| IBIS file stm32u575_585_ufbga169.ibs
[IBIS ver] 4.2
[File name] stm32u575_585_ufbga169.ibs
[File Rev] 1.0
[Date]   06-08-2021
[Source] Data Created at STMicroelectronics
[Notes]  File originated from ELDO simulations.
[Disclaimer]  This information is for modeling purpose only and is
   not guaranted. The information is subject to change without
   notice.
[Copyright] Copyright 2021 STMicroelectronics Inc.
|   Component stm32u575_585_ufbga169
[Component] stm32u575_585_ufbga169
[Manufacturer] STMicroelectronics
[Package]
| variable   typ   min   max
R_pkg   0   NA   NA
L_pkg   0   NA   NA
C_pkg   0   NA   NA
[Pin]   signal_name   model_name   R_pin   L_pin   C_pin   | Comment
A1 PE2 io8_100m_hslv_ft
A10 PA15 nc
A11 VDD POWER
A12 PI1 io8_100m_hslv_ft
A13 PH15 io8_100m_hslv_ft
A2 PI6 io8_166m_hslv_ft
A3 VDD POWER
A4 VCAP POWER
A5 PG15 io8_100m_hslv_ft
A6 VDDIO2 POWER
A7 PG9 io8_100m_hslv_ft
A8 VDD POWER
A9 PC11 io8_100m_hslv_ft
B1 VDD POWER
B10 PI4 io8_100m_ft
B11 VSS GND
B12 PI0 io8_100m_hslv_ft
B13 PH12 io8_100m_hslv_ft
B2 VSS GND
B3 PI5 io8_100m_hslv_ft
B4 VSS GND
B5 PB6 io8_100m_i2c_ft
B6 PB4 io8_100m_i2c_ft
B7 PD6 io8_166m_hslv_ft
B8 VSS GND
B9 PD0 io8_100m_hslv_ft
C1 VBAT POWER
C10 PA14 io8_100m_ft
C11 PH14 io8_100m_ft
C12 PH13 io8_100m_ft
C13 PH10 io8_100m_hslv_ft
C2 PE4 io8_100m_hslv_tamp_ft
C3 PI7 io8_166m_hslv_ft
C4 PE1 io8_100m_hslv_ft
C5 PH3-BOOT0 io8_100m_ft
C6 PB5 io8_166m_hslv_ft
C7 PG10 io8_100m_hslv_ft
C8 PD4 io8_100m_hslv_ft
C9 PC10 io8_100m_ft
D1 PC14-OSC32_IN io8_100m_ft
D10 PI3 io8_100m_hslv_ft
D11 PI2 io8_166m_hslv_ft
D12 PH8 io8_100m_hslv_ft
D13 VDD POWER
D2 PE5 io8_100m_hslv_tamp_ft
D3 PE3 io8_100m_hslv_tamp_ft
D4 PE0 io8_100m_hslv_ft
D5 PB9 io8_100m_i2c_ft
D6 PB3 io8_100m_i2c_ft
D7 PD7 io8_100m_hslv_ft
D8 PD3 io8_166m_hslv_ft
D9 PH11 io8_100m_hslv_ft
E1 PC15-OSC32_OUT io8_100m_ft
E10 PH4 io8_100m_hslv_ft
E11 PH6 io8_166m_hslv_ft
E12 VSS GND
E13 VDDUSB POWER
E2 PF0 io8_100m_hslv_ft
E3 PC13 io8_100m_ft_v33
E4 PE6 io8_100m_hslv_tamp_ft
E5 PB8 io8_100m_i2c_ft
E6 PG12 io8_100m_hslv_ft
E7 PD5 io8_100m_hslv_ft
E8 PC12 io8_166m_hslv_ft
E9 PH9 io8_100m_hslv_ft
F1 PF8 io8_100m_hslv_ft
F10 PH2 io8_100m_hslv_ft
F11 PA10 io8_100m_usb_id
F12 PA13 io8_100m_ft
F13 PA12 io8_usb_ft
F2 VSS GND
F3 PF1 io8_100m_hslv_ft
F4 PF2 io8_100m_hslv_ft
F5 PB7 io8_166m_hslv_i2c_ft
F6 PD1 io8_100m_hslv_ft
F7 PD2 io8_100m_ft
F8 PH7 io8_166m_hslv_i2c_ft
F9 PH5 io8_100m_i2c_ft
G1 VDD POWER
G10 PC8 io8_100m_ft
G11 PA9 io8_100m_usb_vbus_ft
G12 PC7 io8_100m_ft
G13 PA11 io8_usb_ft
G2 PF7 io8_100m_hslv_ft
G3 PF9 io8_100m_hslv_ft
G4 PF5 io8_166m_hslv_ft
G5 PF3 io8_100m_hslv_ft
G6 PF4 io8_166m_hslv_ft
G7 PA8 io8_166m_hslv_ft
G8 PG7 io8_100m_hslv_ft
G9 PC9 io8_100m_ft
H1 PH0-OSC_IN io8_100m_ft
H10 PG6 io8_100m_hslv_ft
H11 PG4 io8_100m_hslv_ft
H12 VDDIO2 POWER
H13 PC6 io8_100m_ft
H2 VSS GND
H3 NRST nc
H4 PF10 io8_166m_hslv_ft
H5 OPAMP2_VINM nc
H6 PF6 io8_100m_hslv_ft
H7 PG1 io8_100m_hslv_ft
H8 PE10 io8_166m_hslv_ft
H9 PG8 io8_100m_i2c_ft
J1 PH1-OSC_OUT io8_100m_ft
J10 PD14 io8_100m_hslv_ft
J11 PD15 io8_100m_hslv_ft
J12 VSS GND
J13 VDD POWER
J2 PC0 io8_100m_hslv_ft
J3 PC1 io8_166m_hslv_i2c_ft
J4 PC2 io8_100m_hslv_ft
J5 PA7 io8_100m_hslv_ft
J6 PG0 io8_100m_hslv_ft
J7 PE9 io8_166m_hslv_ft
J8 PG3 io8_100m_hslv_ft
J9 PG5 io8_100m_hslv_ft
K1 PC3 io8_100m_hslv_ft
K10 PD12 io8_100m_hslv_ft
K11 PD10 io8_100m_hslv_ft
K12 PD13 io8_100m_hslv_ft
K13 PG2 io8_100m_hslv_ft
K2 VSSA GND
K3 PA0 io8_100m_hslv_tamp_ft
K4 PA5 io8_100m_ft
K5 PB0 io8_100m_hslv_ft
K6 PF12 io8_100m_hslv_ft
K7 PE8 io8_100m_hslv_ft
K8 PE14 io8_100m_hslv_ft
K9 PB10 io8_166m_hslv_i2c_ft
L1 VREF+ POWER
L10 PB12 io8_166m_hslv_ft
L11 PB15 nc
L12 PD8 io8_100m_hslv_ft
L13 PD9 io8_100m_hslv_ft
L2 VDDA POWER
L3 PA1 io8_100m_hslv_tamp_ft
L4 PC4 io8_100m_hslv_ft
L5 PB2 io8_100m_hslv_tamp_ft
L6 PF14 io8_100m_hslv_ft
L7 PE7 io8_100m_hslv_ft
L8 PE13 io8_100m_hslv_ft
L9 PB11 io8_100m_hslv_ft
M1 OPAMP1_VINM nc
M10 PG11 io8_100m_hslv_ft
M11 VSS GND
M12 PB14 io8_100m_i2c_ft
M13 PD11 io8_100m_hslv_ft
M2 PA2 io8_100m_hslv_ft
M3 VSS GND
M4 PC5 io8_100m_tamp_ft
M5 PF11 io8_166m_hslv_ft
M6 PF13 io8_100m_hslv_ft
M7 VSS GND
M8 PE11 io8_100m_hslv_ft
M9 PE15 io8_100m_hslv_ft
N1 PA4 io8_100m_hslv_ft
N10 PG13 io8_100m_hslv_ft
N11 VCAP POWER
N12 VDD POWER
N13 PB13 io8_100m_i2c_ft
N2 PA3 io8_166m_hslv_ft
N3 VDD POWER
N4 PA6 io8_100m_hslv_ft
N5 PB1 io8_100m_hslv_ft
N6 PF15 io8_100m_hslv_ft
N7 VDD POWER
N8 PE12 io8_100m_hslv_ft
N9 PG14 io8_100m_hslv_ft
[Model Selector] io8_100m_ft
io8_100m_ft_hs_1v2  "IO8_FT 100MHz high speed @ 1.2V"
io8_100m_ft_hs_pu_1v2  "IO8_FT 100MHz high speed @ 1.2V pullup"
io8_100m_ft_hs_pd_1v2  "IO8_FT 100MHz high speed @ 1.2V pulldown"
io8_100m_ft_fs_1v2  "IO8_FT 100MHz fast speed @ 1.2V"
io8_100m_ft_fs_pu_1v2  "IO8_FT 100MHz fast speed @ 1.2V pullup"
io8_100m_ft_fs_pd_1v2  "IO8_FT 100MHz fast speed @ 1.2V pulldown"
io8_100m_ft_ms_1v2  "IO8_FT 100MHz med speed @ 1.2V"
io8_100m_ft_ms_pu_1v2  "IO8_FT 100MHz med speed @ 1.2V pullup"
io8_100m_ft_ms_pd_1v2  "IO8_FT 100MHz med speed @ 1.2V pulldown"
io8_100m_ft_ls_1v2  "IO8_FT 100MHz low speed @ 1.2V"
io8_100m_ft_ls_pu_1v2  "IO8_FT 100MHz low speed @ 1.2V pullup"
io8_100m_ft_ls_pd_1v2  "IO8_FT 100MHz low speed @ 1.2V pulldown"
io8_100m_ft_hs_1v8  "IO8_FT 100MHz high speed @ 1.8V"
io8_100m_ft_hs_pu_1v8  "IO8_FT 100MHz high speed @ 1.8V pullup"
io8_100m_ft_hs_pd_1v8  "IO8_FT 100MHz high speed @ 1.8V pulldown"
io8_100m_ft_fs_1v8  "IO8_FT 100MHz fast speed @ 1.8V"
io8_100m_ft_fs_pu_1v8  "IO8_FT 100MHz fast speed @ 1.8V pullup"
io8_100m_ft_fs_pd_1v8  "IO8_FT 100MHz fast speed @ 1.8V pulldown"
io8_100m_ft_ms_1v8  "IO8_FT 100MHz med speed @ 1.8V"
io8_100m_ft_ms_pu_1v8  "IO8_FT 100MHz med speed @ 1.8V pullup"
io8_100m_ft_ms_pd_1v8  "IO8_FT 100MHz med speed @ 1.8V pulldown"
io8_100m_ft_ls_1v8  "IO8_FT 100MHz low speed @ 1.8V"
io8_100m_ft_ls_pu_1v8  "IO8_FT 100MHz low speed @ 1.8V pullup"
io8_100m_ft_ls_pd_1v8  "IO8_FT 100MHz low speed @ 1.8V pulldown"
io8_100m_ft_hs_3v3  "IO8_FT 100MHz high speed @ 3.3V"
io8_100m_ft_hs_pu_3v3  "IO8_FT 100MHz high speed @ 3.3V pullup"
io8_100m_ft_hs_pd_3v3  "IO8_FT 100MHz high speed @ 3.3V pulldown"
io8_100m_ft_fs_3v3  "IO8_FT 100MHz fast speed @ 3.3V"
io8_100m_ft_fs_pu_3v3  "IO8_FT 100MHz fast speed @ 3.3V pullup"
io8_100m_ft_fs_pd_3v3  "IO8_FT 100MHz fast speed @ 3.3V pulldown"
io8_100m_ft_ms_3v3  "IO8_FT 100MHz med speed @ 3.3V"
io8_100m_ft_ms_pu_3v3  "IO8_FT 100MHz med speed @ 3.3V pullup"
io8_100m_ft_ms_pd_3v3  "IO8_FT 100MHz med speed @ 3.3V pulldown"
io8_100m_ft_ls_3v3  "IO8_FT 100MHz low speed @ 3.3V"
io8_100m_ft_ls_pu_3v3  "IO8_FT 100MHz low speed @ 3.3V pullup"
io8_100m_ft_ls_pd_3v3  "IO8_FT 100MHz low speed @ 3.3V pulldown"
[Model Selector] io8_100m_hslv_ft
io8_100m_ft_hs_1v2  "IO8_FT 100MHz high speed @ 1.2V"
io8_100m_ft_hs_pu_1v2  "IO8_FT 100MHz high speed @ 1.2V pullup"
io8_100m_ft_hs_pd_1v2  "IO8_FT 100MHz high speed @ 1.2V pulldown"
io8_100m_ft_fs_1v2  "IO8_FT 100MHz fast speed @ 1.2V"
io8_100m_ft_fs_pu_1v2  "IO8_FT 100MHz fast speed @ 1.2V pullup"
io8_100m_ft_fs_pd_1v2  "IO8_FT 100MHz fast speed @ 1.2V pulldown"
io8_100m_ft_ms_1v2  "IO8_FT 100MHz med speed @ 1.2V"
io8_100m_ft_ms_pu_1v2  "IO8_FT 100MHz med speed @ 1.2V pullup"
io8_100m_ft_ms_pd_1v2  "IO8_FT 100MHz med speed @ 1.2V pulldown"
io8_100m_ft_ls_1v2  "IO8_FT 100MHz low speed @ 1.2V"
io8_100m_ft_ls_pu_1v2  "IO8_FT 100MHz low speed @ 1.2V pullup"
io8_100m_ft_ls_pd_1v2  "IO8_FT 100MHz low speed @ 1.2V pulldown"
io8_100m_ft_hs_1v8  "IO8_FT 100MHz high speed @ 1.8V"
io8_100m_ft_hs_pu_1v8  "IO8_FT 100MHz high speed @ 1.8V pullup"
io8_100m_ft_hs_pd_1v8  "IO8_FT 100MHz high speed @ 1.8V pulldown"
io8_100m_ft_fs_1v8  "IO8_FT 100MHz fast speed @ 1.8V"
io8_100m_ft_fs_pu_1v8  "IO8_FT 100MHz fast speed @ 1.8V pullup"
io8_100m_ft_fs_pd_1v8  "IO8_FT 100MHz fast speed @ 1.8V pulldown"
io8_100m_ft_ms_1v8  "IO8_FT 100MHz med speed @ 1.8V"
io8_100m_ft_ms_pu_1v8  "IO8_FT 100MHz med speed @ 1.8V pullup"
io8_100m_ft_ms_pd_1v8  "IO8_FT 100MHz med speed @ 1.8V pulldown"
io8_100m_ft_ls_1v8  "IO8_FT 100MHz low speed @ 1.8V"
io8_100m_ft_ls_pu_1v8  "IO8_FT 100MHz low speed @ 1.8V pullup"
io8_100m_ft_ls_pd_1v8  "IO8_FT 100MHz low speed @ 1.8V pulldown"
io8_100m_ft_hs_3v3  "IO8_FT 100MHz high speed @ 3.3V"
io8_100m_ft_hs_pu_3v3  "IO8_FT 100MHz high speed @ 3.3V pullup"
io8_100m_ft_hs_pd_3v3  "IO8_FT 100MHz high speed @ 3.3V pulldown"
io8_100m_ft_fs_3v3  "IO8_FT 100MHz fast speed @ 3.3V"
io8_100m_ft_fs_pu_3v3  "IO8_FT 100MHz fast speed @ 3.3V pullup"
io8_100m_ft_fs_pd_3v3  "IO8_FT 100MHz fast speed @ 3.3V pulldown"
io8_100m_ft_ms_3v3  "IO8_FT 100MHz med speed @ 3.3V"
io8_100m_ft_ms_pu_3v3  "IO8_FT 100MHz med speed @ 3.3V pullup"
io8_100m_ft_ms_pd_3v3  "IO8_FT 100MHz med speed @ 3.3V pulldown"
io8_100m_ft_ls_3v3  "IO8_FT 100MHz low speed @ 3.3V"
io8_100m_ft_ls_pu_3v3  "IO8_FT 100MHz low speed @ 3.3V pullup"
io8_100m_ft_ls_pd_3v3  "IO8_FT 100MHz low speed @ 3.3V pulldown"
io8_100m_hslv_ft_hs_1v2  "IO8_FT 100MHz HSLV high speed @ 1.2V"
io8_100m_hslv_ft_hs_pu_1v2  "IO8_FT 100MHz HSLV high speed @ 1.2V pullup"
io8_100m_hslv_ft_hs_pd_1v2  "IO8_FT 100MHz HSLV high speed @ 1.2V pulldown"
io8_100m_hslv_ft_fs_1v2  "IO8_FT 100MHz HSLV fast speed @ 1.2V"
io8_100m_hslv_ft_fs_pu_1v2  "IO8_FT 100MHz HSLV fast speed @ 1.2V pullup"
io8_100m_hslv_ft_fs_pd_1v2  "IO8_FT 100MHz HSLV fast speed @ 1.2V pulldown"
io8_100m_hslv_ft_ms_1v2  "IO8_FT 100MHz HSLV med speed @ 1.2V"
io8_100m_hslv_ft_ms_pu_1v2  "IO8_FT 100MHz HSLV med speed @ 1.2V pullup"
io8_100m_hslv_ft_ms_pd_1v2  "IO8_FT 100MHz HSLV med speed @ 1.2V pulldown"
io8_100m_hslv_ft_ls_1v2  "IO8_FT 100MHz HSLV low speed @ 1.2V"
io8_100m_hslv_ft_ls_pu_1v2  "IO8_FT 100MHz HSLV low speed @ 1.2V pullup"
io8_100m_hslv_ft_ls_pd_1v2  "IO8_FT 100MHz HSLV low speed @ 1.2V pulldown"
io8_100m_hslv_ft_hs_1v8  "IO8_FT 100MHz HSLV high speed @ 1.8V"
io8_100m_hslv_ft_hs_pu_1v8  "IO8_FT 100MHz HSLV high speed @ 1.8V pullup"
io8_100m_hslv_ft_hs_pd_1v8  "IO8_FT 100MHz HSLV high speed @ 1.8V pulldown"
io8_100m_hslv_ft_fs_1v8  "IO8_FT 100MHz HSLV fast speed @ 1.8V"
io8_100m_hslv_ft_fs_pu_1v8  "IO8_FT 100MHz HSLV fast speed @ 1.8V pullup"
io8_100m_hslv_ft_fs_pd_1v8  "IO8_FT 100MHz HSLV fast speed @ 1.8V pulldown"
io8_100m_hslv_ft_ms_1v8  "IO8_FT 100MHz HSLV med speed @ 1.8V"
io8_100m_hslv_ft_ms_pu_1v8  "IO8_FT 100MHz HSLV med speed @ 1.8V pullup"
io8_100m_hslv_ft_ms_pd_1v8  "IO8_FT 100MHz HSLV med speed @ 1.8V pulldown"
io8_100m_hslv_ft_ls_1v8  "IO8_FT 100MHz HSLV low speed @ 1.8V"
io8_100m_hslv_ft_ls_pu_1v8  "IO8_FT 100MHz HSLV low speed @ 1.8V pullup"
io8_100m_hslv_ft_ls_pd_1v8  "IO8_FT 100MHz HSLV low speed @ 1.8V pulldown"
io8_100m_hslv_ft_hs_2v5  "IO8_FT 100MHz HSLV high speed @ 2.5V"
io8_100m_hslv_ft_hs_pu_2v5  "IO8_FT 100MHz HSLV high speed @ 2.5V pullup"
io8_100m_hslv_ft_hs_pd_2v5  "IO8_FT 100MHz HSLV high speed @ 2.5V pulldown"
io8_100m_hslv_ft_fs_2v5  "IO8_FT 100MHz HSLV fast speed @ 2.5V"
io8_100m_hslv_ft_fs_pu_2v5  "IO8_FT 100MHz HSLV fast speed @ 2.5V pullup"
io8_100m_hslv_ft_fs_pd_2v5  "IO8_FT 100MHz HSLV fast speed @ 2.5V pulldown"
io8_100m_hslv_ft_ms_2v5  "IO8_FT 100MHz HSLV med speed @ 2.5V"
io8_100m_hslv_ft_ms_pu_2v5  "IO8_FT 100MHz HSLV med speed @ 2.5V pullup"
io8_100m_hslv_ft_ms_pd_2v5  "IO8_FT 100MHz HSLV med speed @ 2.5V pulldown"
io8_100m_hslv_ft_ls_2v5  "IO8_FT 100MHz HSLV low speed @ 2.5V"
io8_100m_hslv_ft_ls_pu_2v5  "IO8_FT 100MHz HSLV low speed @ 2.5V pullup"
io8_100m_hslv_ft_ls_pd_2v5  "IO8_FT 100MHz HSLV low speed @ 2.5V pulldown"
[Model Selector] io8_166m_hslv_ft
io8_166m_ft_hs_1v2  "IO8_FT 166MHz high speed @ 1.2V"
io8_166m_ft_hs_pu_1v2  "IO8_FT 166MHz high speed @ 1.2V pullup"
io8_166m_ft_hs_pd_1v2  "IO8_FT 166MHz high speed @ 1.2V pulldown"
io8_166m_ft_fs_1v2  "IO8_FT 166MHz fast speed @ 1.2V"
io8_166m_ft_fs_pu_1v2  "IO8_FT 166MHz fast speed @ 1.2V pullup"
io8_166m_ft_fs_pd_1v2  "IO8_FT 166MHz fast speed @ 1.2V pulldown"
io8_166m_ft_ms_1v2  "IO8_FT 166MHz med speed @ 1.2V"
io8_166m_ft_ms_pu_1v2  "IO8_FT 166MHz med speed @ 1.2V pullup"
io8_166m_ft_ms_pd_1v2  "IO8_FT 166MHz med speed @ 1.2V pulldown"
io8_166m_ft_ls_1v2  "IO8_FT 166MHz low speed @ 1.2V"
io8_166m_ft_ls_pu_1v2  "IO8_FT 166MHz low speed @ 1.2V pullup"
io8_166m_ft_ls_pd_1v2  "IO8_FT 166MHz low speed @ 1.2V pulldown"
io8_166m_ft_hs_1v8  "IO8_FT 166MHz high speed @ 1.8V"
io8_166m_ft_hs_pu_1v8  "IO8_FT 166MHz high speed @ 1.8V pullup"
io8_166m_ft_hs_pd_1v8  "IO8_FT 166MHz high speed @ 1.8V pulldown"
io8_166m_ft_fs_1v8  "IO8_FT 166MHz fast speed @ 1.8V"
io8_166m_ft_fs_pu_1v8  "IO8_FT 166MHz fast speed @ 1.8V pullup"
io8_166m_ft_fs_pd_1v8  "IO8_FT 166MHz fast speed @ 1.8V pulldown"
io8_166m_ft_ms_1v8  "IO8_FT 166MHz med speed @ 1.8V"
io8_166m_ft_ms_pu_1v8  "IO8_FT 166MHz med speed @ 1.8V pullup"
io8_166m_ft_ms_pd_1v8  "IO8_FT 166MHz med speed @ 1.8V pulldown"
io8_166m_ft_ls_1v8  "IO8_FT 166MHz low speed @ 1.8V"
io8_166m_ft_ls_pu_1v8  "IO8_FT 166MHz low speed @ 1.8V pullup"
io8_166m_ft_ls_pd_1v8  "IO8_FT 166MHz low speed @ 1.8V pulldown"
io8_166m_ft_hs_3v3  "IO8_FT 166MHz high speed @ 3.3V"
io8_166m_ft_hs_pu_3v3  "IO8_FT 166MHz high speed @ 3.3V pullup"
io8_166m_ft_hs_pd_3v3  "IO8_FT 166MHz high speed @ 3.3V pulldown"
io8_166m_ft_fs_3v3  "IO8_FT 166MHz fast speed @ 3.3V"
io8_166m_ft_fs_pu_3v3  "IO8_FT 166MHz fast speed @ 3.3V pullup"
io8_166m_ft_fs_pd_3v3  "IO8_FT 166MHz fast speed @ 3.3V pulldown"
io8_166m_ft_ms_3v3  "IO8_FT 166MHz med speed @ 3.3V"
io8_166m_ft_ms_pu_3v3  "IO8_FT 166MHz med speed @ 3.3V pullup"
io8_166m_ft_ms_pd_3v3  "IO8_FT 166MHz med speed @ 3.3V pulldown"
io8_166m_ft_ls_3v3  "IO8_FT 166MHz low speed @ 3.3V"
io8_166m_ft_ls_pu_3v3  "IO8_FT 166MHz low speed @ 3.3V pullup"
io8_166m_ft_ls_pd_3v3  "IO8_FT 166MHz low speed @ 3.3V pulldown"
io8_166m_hslv_ft_hs_1v2  "IO8_FT 166MHz HSLV high speed @ 1.2V"
io8_166m_hslv_ft_hs_pu_1v2  "IO8_FT 166MHz HSLV high speed @ 1.2V pullup"
io8_166m_hslv_ft_hs_pd_1v2  "IO8_FT 166MHz HSLV high speed @ 1.2V pulldown"
io8_166m_hslv_ft_fs_1v2  "IO8_FT 166MHz HSLV fast speed @ 1.2V"
io8_166m_hslv_ft_fs_pu_1v2  "IO8_FT 166MHz HSLV fast speed @ 1.2V pullup"
io8_166m_hslv_ft_fs_pd_1v2  "IO8_FT 166MHz HSLV fast speed @ 1.2V pulldown"
io8_166m_hslv_ft_ms_1v2  "IO8_FT 166MHz HSLV med speed @ 1.2V"
io8_166m_hslv_ft_ms_pu_1v2  "IO8_FT 166MHz HSLV med speed @ 1.2V pullup"
io8_166m_hslv_ft_ms_pd_1v2  "IO8_FT 166MHz HSLV med speed @ 1.2V pulldown"
io8_166m_hslv_ft_ls_1v2  "IO8_FT 166MHz HSLV low speed @ 1.2V"
io8_166m_hslv_ft_ls_pu_1v2  "IO8_FT 166MHz HSLV low speed @ 1.2V pullup"
io8_166m_hslv_ft_ls_pd_1v2  "IO8_FT 166MHz HSLV low speed @ 1.2V pulldown"
io8_166m_hslv_ft_hs_1v8  "IO8_FT 166MHz HSLV high speed @ 1.8V"
io8_166m_hslv_ft_hs_pu_1v8  "IO8_FT 166MHz HSLV high speed @ 1.8V pullup"
io8_166m_hslv_ft_hs_pd_1v8  "IO8_FT 166MHz HSLV high speed @ 1.8V pulldown"
io8_166m_hslv_ft_fs_1v8  "IO8_FT 166MHz HSLV fast speed @ 1.8V"
io8_166m_hslv_ft_fs_pu_1v8  "IO8_FT 166MHz HSLV fast speed @ 1.8V pullup"
io8_166m_hslv_ft_fs_pd_1v8  "IO8_FT 166MHz HSLV fast speed @ 1.8V pulldown"
io8_166m_hslv_ft_ms_1v8  "IO8_FT 166MHz HSLV med speed @ 1.8V"
io8_166m_hslv_ft_ms_pu_1v8  "IO8_FT 166MHz HSLV med speed @ 1.8V pullup"
io8_166m_hslv_ft_ms_pd_1v8  "IO8_FT 166MHz HSLV med speed @ 1.8V pulldown"
io8_166m_hslv_ft_ls_1v8  "IO8_FT 166MHz HSLV low speed @ 1.8V"
io8_166m_hslv_ft_ls_pu_1v8  "IO8_FT 166MHz HSLV low speed @ 1.8V pullup"
io8_166m_hslv_ft_ls_pd_1v8  "IO8_FT 166MHz HSLV low speed @ 1.8V pulldown"
io8_166m_hslv_ft_hs_2v5  "IO8_FT 166MHz HSLV high speed @ 2.5V"
io8_166m_hslv_ft_hs_pu_2v5  "IO8_FT 166MHz HSLV high speed @ 2.5V pullup"
io8_166m_hslv_ft_hs_pd_2v5  "IO8_FT 166MHz HSLV high speed @ 2.5V pulldown"
io8_166m_hslv_ft_fs_2v5  "IO8_FT 166MHz HSLV fast speed @ 2.5V"
io8_166m_hslv_ft_fs_pu_2v5  "IO8_FT 166MHz HSLV fast speed @ 2.5V pullup"
io8_166m_hslv_ft_fs_pd_2v5  "IO8_FT 166MHz HSLV fast speed @ 2.5V pulldown"
io8_166m_hslv_ft_ms_2v5  "IO8_FT 166MHz HSLV med speed @ 2.5V"
io8_166m_hslv_ft_ms_pu_2v5  "IO8_FT 166MHz HSLV med speed @ 2.5V pullup"
io8_166m_hslv_ft_ms_pd_2v5  "IO8_FT 166MHz HSLV med speed @ 2.5V pulldown"
io8_166m_hslv_ft_ls_2v5  "IO8_FT 166MHz HSLV low speed @ 2.5V"
io8_166m_hslv_ft_ls_pu_2v5  "IO8_FT 166MHz HSLV low speed @ 2.5V pullup"
io8_166m_hslv_ft_ls_pd_2v5  "IO8_FT 166MHz HSLV low speed @ 2.5V pulldown"
[Model Selector] io8_100m_ft_v33
io8_ft_v33_hs_1v2  "IO8_FT_V33 high speed @ 1.2V"
io8_ft_v33_hs_pu_1v2  "IO8_FT_V33 high speed @ 1.2V pullup"
io8_ft_v33_hs_pd_1v2  "IO8_FT_V33 high speed @ 1.2V pulldown"
io8_ft_v33_fs_1v2  "IO8_FT_V33 fast speed @ 1.2V"
io8_ft_v33_fs_pu_1v2  "IO8_FT_V33 fast speed @ 1.2V pullup"
io8_ft_v33_fs_pd_1v2  "IO8_FT_V33 fast speed @ 1.2V pulldown"
io8_ft_v33_ms_1v2  "IO8_FT_V33 med speed @ 1.2V"
io8_ft_v33_ms_pu_1v2  "IO8_FT_V33 med speed @ 1.2V pullup"
io8_ft_v33_ms_pd_1v2  "IO8_FT_V33 med speed @ 1.2V pulldown"
io8_ft_v33_ls_1v2  "IO8_FT_V33 low speed @ 1.2V"
io8_ft_v33_ls_pu_1v2  "IO8_FT_V33 low speed @ 1.2V pullup"
io8_ft_v33_ls_pd_1v2  "IO8_FT_V33 low speed @ 1.2V pulldown"
io8_ft_v33_hs_1v8  "IO8_FT_V33 high speed @ 1.8V"
io8_ft_v33_hs_pu_1v8  "IO8_FT_V33 high speed @ 1.8V pullup"
io8_ft_v33_hs_pd_1v8  "IO8_FT_V33 high speed @ 1.8V pulldown"
io8_ft_v33_fs_1v8  "IO8_FT_V33 fast speed @ 1.8V"
io8_ft_v33_fs_pu_1v8  "IO8_FT_V33 fast speed @ 1.8V pullup"
io8_ft_v33_fs_pd_1v8  "IO8_FT_V33 fast speed @ 1.8V pulldown"
io8_ft_v33_ms_1v8  "IO8_FT_V33 med speed @ 1.8V"
io8_ft_v33_ms_pu_1v8  "IO8_FT_V33 med speed @ 1.8V pullup"
io8_ft_v33_ms_pd_1v8  "IO8_FT_V33 med speed @ 1.8V pulldown"
io8_ft_v33_ls_1v8  "IO8_FT_V33 low speed @ 1.8V"
io8_ft_v33_ls_pu_1v8  "IO8_FT_V33 low speed @ 1.8V pullup"
io8_ft_v33_ls_pd_1v8  "IO8_FT_V33 low speed @ 1.8V pulldown"
io8_ft_v33_hs_3v3  "IO8_FT_V33 high speed @ 3.3V"
io8_ft_v33_hs_pu_3v3  "IO8_FT_V33 high speed @ 3.3V pullup"
io8_ft_v33_hs_pd_3v3  "IO8_FT_V33 high speed @ 3.3V pulldown"
io8_ft_v33_fs_3v3  "IO8_FT_V33 fast speed @ 3.3V"
io8_ft_v33_fs_pu_3v3  "IO8_FT_V33 fast speed @ 3.3V pullup"
io8_ft_v33_fs_pd_3v3  "IO8_FT_V33 fast speed @ 3.3V pulldown"
io8_ft_v33_ms_3v3  "IO8_FT_V33 med speed @ 3.3V"
io8_ft_v33_ms_pu_3v3  "IO8_FT_V33 med speed @ 3.3V pullup"
io8_ft_v33_ms_pd_3v3  "IO8_FT_V33 med speed @ 3.3V pulldown"
io8_ft_v33_ls_3v3  "IO8_FT_V33 low speed @ 3.3V"
io8_ft_v33_ls_pu_3v3  "IO8_FT_V33 low speed @ 3.3V pullup"
io8_ft_v33_ls_pd_3v3  "IO8_FT_V33 low speed @ 3.3V pulldown"
[Model Selector] io8_100m_tamp_ft
io8_100m_ft_hs_1v2  "IO8_FT 100MHz high speed @ 1.2V"
io8_100m_ft_hs_pu_1v2  "IO8_FT 100MHz high speed @ 1.2V pullup"
io8_100m_ft_hs_pd_1v2  "IO8_FT 100MHz high speed @ 1.2V pulldown"
io8_100m_ft_fs_1v2  "IO8_FT 100MHz fast speed @ 1.2V"
io8_100m_ft_fs_pu_1v2  "IO8_FT 100MHz fast speed @ 1.2V pullup"
io8_100m_ft_fs_pd_1v2  "IO8_FT 100MHz fast speed @ 1.2V pulldown"
io8_100m_ft_ms_1v2  "IO8_FT 100MHz med speed @ 1.2V"
io8_100m_ft_ms_pu_1v2  "IO8_FT 100MHz med speed @ 1.2V pullup"
io8_100m_ft_ms_pd_1v2  "IO8_FT 100MHz med speed @ 1.2V pulldown"
io8_100m_ft_ls_1v2  "IO8_FT 100MHz low speed @ 1.2V"
io8_100m_ft_ls_pu_1v2  "IO8_FT 100MHz low speed @ 1.2V pullup"
io8_100m_ft_ls_pd_1v2  "IO8_FT 100MHz low speed @ 1.2V pulldown"
io8_100m_ft_hs_1v8  "IO8_FT 100MHz high speed @ 1.8V"
io8_100m_ft_hs_pu_1v8  "IO8_FT 100MHz high speed @ 1.8V pullup"
io8_100m_ft_hs_pd_1v8  "IO8_FT 100MHz high speed @ 1.8V pulldown"
io8_100m_ft_fs_1v8  "IO8_FT 100MHz fast speed @ 1.8V"
io8_100m_ft_fs_pu_1v8  "IO8_FT 100MHz fast speed @ 1.8V pullup"
io8_100m_ft_fs_pd_1v8  "IO8_FT 100MHz fast speed @ 1.8V pulldown"
io8_100m_ft_ms_1v8  "IO8_FT 100MHz med speed @ 1.8V"
io8_100m_ft_ms_pu_1v8  "IO8_FT 100MHz med speed @ 1.8V pullup"
io8_100m_ft_ms_pd_1v8  "IO8_FT 100MHz med speed @ 1.8V pulldown"
io8_100m_ft_ls_1v8  "IO8_FT 100MHz low speed @ 1.8V"
io8_100m_ft_ls_pu_1v8  "IO8_FT 100MHz low speed @ 1.8V pullup"
io8_100m_ft_ls_pd_1v8  "IO8_FT 100MHz low speed @ 1.8V pulldown"
io8_100m_ft_hs_3v3  "IO8_FT 100MHz high speed @ 3.3V"
io8_100m_ft_hs_pu_3v3  "IO8_FT 100MHz high speed @ 3.3V pullup"
io8_100m_ft_hs_pd_3v3  "IO8_FT 100MHz high speed @ 3.3V pulldown"
io8_100m_ft_fs_3v3  "IO8_FT 100MHz fast speed @ 3.3V"
io8_100m_ft_fs_pu_3v3  "IO8_FT 100MHz fast speed @ 3.3V pullup"
io8_100m_ft_fs_pd_3v3  "IO8_FT 100MHz fast speed @ 3.3V pulldown"
io8_100m_ft_ms_3v3  "IO8_FT 100MHz med speed @ 3.3V"
io8_100m_ft_ms_pu_3v3  "IO8_FT 100MHz med speed @ 3.3V pullup"
io8_100m_ft_ms_pd_3v3  "IO8_FT 100MHz med speed @ 3.3V pulldown"
io8_100m_ft_ls_3v3  "IO8_FT 100MHz low speed @ 3.3V"
io8_100m_ft_ls_pu_3v3  "IO8_FT 100MHz low speed @ 3.3V pullup"
io8_100m_ft_ls_pd_3v3  "IO8_FT 100MHz low speed @ 3.3V pulldown"
io8_ft_v33_hs_1v2  "IO8_FT_V33 high speed @ 1.2V"
io8_ft_v33_hs_pu_1v2  "IO8_FT_V33 high speed @ 1.2V pullup"
io8_ft_v33_hs_pd_1v2  "IO8_FT_V33 high speed @ 1.2V pulldown"
io8_ft_v33_fs_1v2  "IO8_FT_V33 fast speed @ 1.2V"
io8_ft_v33_fs_pu_1v2  "IO8_FT_V33 fast speed @ 1.2V pullup"
io8_ft_v33_fs_pd_1v2  "IO8_FT_V33 fast speed @ 1.2V pulldown"
io8_ft_v33_ms_1v2  "IO8_FT_V33 med speed @ 1.2V"
io8_ft_v33_ms_pu_1v2  "IO8_FT_V33 med speed @ 1.2V pullup"
io8_ft_v33_ms_pd_1v2  "IO8_FT_V33 med speed @ 1.2V pulldown"
io8_ft_v33_ls_1v2  "IO8_FT_V33 low speed @ 1.2V"
io8_ft_v33_ls_pu_1v2  "IO8_FT_V33 low speed @ 1.2V pullup"
io8_ft_v33_ls_pd_1v2  "IO8_FT_V33 low speed @ 1.2V pulldown"
io8_ft_v33_hs_1v8  "IO8_FT_V33 high speed @ 1.8V"
io8_ft_v33_hs_pu_1v8  "IO8_FT_V33 high speed @ 1.8V pullup"
io8_ft_v33_hs_pd_1v8  "IO8_FT_V33 high speed @ 1.8V pulldown"
io8_ft_v33_fs_1v8  "IO8_FT_V33 fast speed @ 1.8V"
io8_ft_v33_fs_pu_1v8  "IO8_FT_V33 fast speed @ 1.8V pullup"
io8_ft_v33_fs_pd_1v8  "IO8_FT_V33 fast speed @ 1.8V pulldown"
io8_ft_v33_ms_1v8  "IO8_FT_V33 med speed @ 1.8V"
io8_ft_v33_ms_pu_1v8  "IO8_FT_V33 med speed @ 1.8V pullup"
io8_ft_v33_ms_pd_1v8  "IO8_FT_V33 med speed @ 1.8V pulldown"
io8_ft_v33_ls_1v8  "IO8_FT_V33 low speed @ 1.8V"
io8_ft_v33_ls_pu_1v8  "IO8_FT_V33 low speed @ 1.8V pullup"
io8_ft_v33_ls_pd_1v8  "IO8_FT_V33 low speed @ 1.8V pulldown"
io8_ft_v33_hs_3v3  "IO8_FT_V33 high speed @ 3.3V"
io8_ft_v33_hs_pu_3v3  "IO8_FT_V33 high speed @ 3.3V pullup"
io8_ft_v33_hs_pd_3v3  "IO8_FT_V33 high speed @ 3.3V pulldown"
io8_ft_v33_fs_3v3  "IO8_FT_V33 fast speed @ 3.3V"
io8_ft_v33_fs_pu_3v3  "IO8_FT_V33 fast speed @ 3.3V pullup"
io8_ft_v33_fs_pd_3v3  "IO8_FT_V33 fast speed @ 3.3V pulldown"
io8_ft_v33_ms_3v3  "IO8_FT_V33 med speed @ 3.3V"
io8_ft_v33_ms_pu_3v3  "IO8_FT_V33 med speed @ 3.3V pullup"
io8_ft_v33_ms_pd_3v3  "IO8_FT_V33 med speed @ 3.3V pulldown"
io8_ft_v33_ls_3v3  "IO8_FT_V33 low speed @ 3.3V"
io8_ft_v33_ls_pu_3v3  "IO8_FT_V33 low speed @ 3.3V pullup"
io8_ft_v33_ls_pd_3v3  "IO8_FT_V33 low speed @ 3.3V pulldown"
[Model Selector] io8_100m_hslv_tamp_ft
io8_100m_ft_hs_1v2  "IO8_FT 100MHz high speed @ 1.2V"
io8_100m_ft_hs_pu_1v2  "IO8_FT 100MHz high speed @ 1.2V pullup"
io8_100m_ft_hs_pd_1v2  "IO8_FT 100MHz high speed @ 1.2V pulldown"
io8_100m_ft_fs_1v2  "IO8_FT 100MHz fast speed @ 1.2V"
io8_100m_ft_fs_pu_1v2  "IO8_FT 100MHz fast speed @ 1.2V pullup"
io8_100m_ft_fs_pd_1v2  "IO8_FT 100MHz fast speed @ 1.2V pulldown"
io8_100m_ft_ms_1v2  "IO8_FT 100MHz med speed @ 1.2V"
io8_100m_ft_ms_pu_1v2  "IO8_FT 100MHz med speed @ 1.2V pullup"
io8_100m_ft_ms_pd_1v2  "IO8_FT 100MHz med speed @ 1.2V pulldown"
io8_100m_ft_ls_1v2  "IO8_FT 100MHz low speed @ 1.2V"
io8_100m_ft_ls_pu_1v2  "IO8_FT 100MHz low speed @ 1.2V pullup"
io8_100m_ft_ls_pd_1v2  "IO8_FT 100MHz low speed @ 1.2V pulldown"
io8_100m_ft_hs_1v8  "IO8_FT 100MHz high speed @ 1.8V"
io8_100m_ft_hs_pu_1v8  "IO8_FT 100MHz high speed @ 1.8V pullup"
io8_100m_ft_hs_pd_1v8  "IO8_FT 100MHz high speed @ 1.8V pulldown"
io8_100m_ft_fs_1v8  "IO8_FT 100MHz fast speed @ 1.8V"
io8_100m_ft_fs_pu_1v8  "IO8_FT 100MHz fast speed @ 1.8V pullup"
io8_100m_ft_fs_pd_1v8  "IO8_FT 100MHz fast speed @ 1.8V pulldown"
io8_100m_ft_ms_1v8  "IO8_FT 100MHz med speed @ 1.8V"
io8_100m_ft_ms_pu_1v8  "IO8_FT 100MHz med speed @ 1.8V pullup"
io8_100m_ft_ms_pd_1v8  "IO8_FT 100MHz med speed @ 1.8V pulldown"
io8_100m_ft_ls_1v8  "IO8_FT 100MHz low speed @ 1.8V"
io8_100m_ft_ls_pu_1v8  "IO8_FT 100MHz low speed @ 1.8V pullup"
io8_100m_ft_ls_pd_1v8  "IO8_FT 100MHz low speed @ 1.8V pulldown"
io8_100m_ft_hs_3v3  "IO8_FT 100MHz high speed @ 3.3V"
io8_100m_ft_hs_pu_3v3  "IO8_FT 100MHz high speed @ 3.3V pullup"
io8_100m_ft_hs_pd_3v3  "IO8_FT 100MHz high speed @ 3.3V pulldown"
io8_100m_ft_fs_3v3  "IO8_FT 100MHz fast speed @ 3.3V"
io8_100m_ft_fs_pu_3v3  "IO8_FT 100MHz fast speed @ 3.3V pullup"
io8_100m_ft_fs_pd_3v3  "IO8_FT 100MHz fast speed @ 3.3V pulldown"
io8_100m_ft_ms_3v3  "IO8_FT 100MHz med speed @ 3.3V"
io8_100m_ft_ms_pu_3v3  "IO8_FT 100MHz med speed @ 3.3V pullup"
io8_100m_ft_ms_pd_3v3  "IO8_FT 100MHz med speed @ 3.3V pulldown"
io8_100m_ft_ls_3v3  "IO8_FT 100MHz low speed @ 3.3V"
io8_100m_ft_ls_pu_3v3  "IO8_FT 100MHz low speed @ 3.3V pullup"
io8_100m_ft_ls_pd_3v3  "IO8_FT 100MHz low speed @ 3.3V pulldown"
io8_100m_hslv_ft_hs_1v2  "IO8_FT 100MHz HSLV high speed @ 1.2V"
io8_100m_hslv_ft_hs_pu_1v2  "IO8_FT 100MHz HSLV high speed @ 1.2V pullup"
io8_100m_hslv_ft_hs_pd_1v2  "IO8_FT 100MHz HSLV high speed @ 1.2V pulldown"
io8_100m_hslv_ft_fs_1v2  "IO8_FT 100MHz HSLV fast speed @ 1.2V"
io8_100m_hslv_ft_fs_pu_1v2  "IO8_FT 100MHz HSLV fast speed @ 1.2V pullup"
io8_100m_hslv_ft_fs_pd_1v2  "IO8_FT 100MHz HSLV fast speed @ 1.2V pulldown"
io8_100m_hslv_ft_ms_1v2  "IO8_FT 100MHz HSLV med speed @ 1.2V"
io8_100m_hslv_ft_ms_pu_1v2  "IO8_FT 100MHz HSLV med speed @ 1.2V pullup"
io8_100m_hslv_ft_ms_pd_1v2  "IO8_FT 100MHz HSLV med speed @ 1.2V pulldown"
io8_100m_hslv_ft_ls_1v2  "IO8_FT 100MHz HSLV low speed @ 1.2V"
io8_100m_hslv_ft_ls_pu_1v2  "IO8_FT 100MHz HSLV low speed @ 1.2V pullup"
io8_100m_hslv_ft_ls_pd_1v2  "IO8_FT 100MHz HSLV low speed @ 1.2V pulldown"
io8_100m_hslv_ft_hs_1v8  "IO8_FT 100MHz HSLV high speed @ 1.8V"
io8_100m_hslv_ft_hs_pu_1v8  "IO8_FT 100MHz HSLV high speed @ 1.8V pullup"
io8_100m_hslv_ft_hs_pd_1v8  "IO8_FT 100MHz HSLV high speed @ 1.8V pulldown"
io8_100m_hslv_ft_fs_1v8  "IO8_FT 100MHz HSLV fast speed @ 1.8V"
io8_100m_hslv_ft_fs_pu_1v8  "IO8_FT 100MHz HSLV fast speed @ 1.8V pullup"
io8_100m_hslv_ft_fs_pd_1v8  "IO8_FT 100MHz HSLV fast speed @ 1.8V pulldown"
io8_100m_hslv_ft_ms_1v8  "IO8_FT 100MHz HSLV med speed @ 1.8V"
io8_100m_hslv_ft_ms_pu_1v8  "IO8_FT 100MHz HSLV med speed @ 1.8V pullup"
io8_100m_hslv_ft_ms_pd_1v8  "IO8_FT 100MHz HSLV med speed @ 1.8V pulldown"
io8_100m_hslv_ft_ls_1v8  "IO8_FT 100MHz HSLV low speed @ 1.8V"
io8_100m_hslv_ft_ls_pu_1v8  "IO8_FT 100MHz HSLV low speed @ 1.8V pullup"
io8_100m_hslv_ft_ls_pd_1v8  "IO8_FT 100MHz HSLV low speed @ 1.8V pulldown"
io8_100m_hslv_ft_hs_2v5  "IO8_FT 100MHz HSLV high speed @ 2.5V"
io8_100m_hslv_ft_hs_pu_2v5  "IO8_FT 100MHz HSLV high speed @ 2.5V pullup"
io8_100m_hslv_ft_hs_pd_2v5  "IO8_FT 100MHz HSLV high speed @ 2.5V pulldown"
io8_100m_hslv_ft_fs_2v5  "IO8_FT 100MHz HSLV fast speed @ 2.5V"
io8_100m_hslv_ft_fs_pu_2v5  "IO8_FT 100MHz HSLV fast speed @ 2.5V pullup"
io8_100m_hslv_ft_fs_pd_2v5  "IO8_FT 100MHz HSLV fast speed @ 2.5V pulldown"
io8_100m_hslv_ft_ms_2v5  "IO8_FT 100MHz HSLV med speed @ 2.5V"
io8_100m_hslv_ft_ms_pu_2v5  "IO8_FT 100MHz HSLV med speed @ 2.5V pullup"
io8_100m_hslv_ft_ms_pd_2v5  "IO8_FT 100MHz HSLV med speed @ 2.5V pulldown"
io8_100m_hslv_ft_ls_2v5  "IO8_FT 100MHz HSLV low speed @ 2.5V"
io8_100m_hslv_ft_ls_pu_2v5  "IO8_FT 100MHz HSLV low speed @ 2.5V pullup"
io8_100m_hslv_ft_ls_pd_2v5  "IO8_FT 100MHz HSLV low speed @ 2.5V pulldown"
io8_ft_v33_hs_1v2  "IO8_FT_V33 high speed @ 1.2V"
io8_ft_v33_hs_pu_1v2  "IO8_FT_V33 high speed @ 1.2V pullup"
io8_ft_v33_hs_pd_1v2  "IO8_FT_V33 high speed @ 1.2V pulldown"
io8_ft_v33_fs_1v2  "IO8_FT_V33 fast speed @ 1.2V"
io8_ft_v33_fs_pu_1v2  "IO8_FT_V33 fast speed @ 1.2V pullup"
io8_ft_v33_fs_pd_1v2  "IO8_FT_V33 fast speed @ 1.2V pulldown"
io8_ft_v33_ms_1v2  "IO8_FT_V33 med speed @ 1.2V"
io8_ft_v33_ms_pu_1v2  "IO8_FT_V33 med speed @ 1.2V pullup"
io8_ft_v33_ms_pd_1v2  "IO8_FT_V33 med speed @ 1.2V pulldown"
io8_ft_v33_ls_1v2  "IO8_FT_V33 low speed @ 1.2V"
io8_ft_v33_ls_pu_1v2  "IO8_FT_V33 low speed @ 1.2V pullup"
io8_ft_v33_ls_pd_1v2  "IO8_FT_V33 low speed @ 1.2V pulldown"
io8_ft_v33_hs_1v8  "IO8_FT_V33 high speed @ 1.8V"
io8_ft_v33_hs_pu_1v8  "IO8_FT_V33 high speed @ 1.8V pullup"
io8_ft_v33_hs_pd_1v8  "IO8_FT_V33 high speed @ 1.8V pulldown"
io8_ft_v33_fs_1v8  "IO8_FT_V33 fast speed @ 1.8V"
io8_ft_v33_fs_pu_1v8  "IO8_FT_V33 fast speed @ 1.8V pullup"
io8_ft_v33_fs_pd_1v8  "IO8_FT_V33 fast speed @ 1.8V pulldown"
io8_ft_v33_ms_1v8  "IO8_FT_V33 med speed @ 1.8V"
io8_ft_v33_ms_pu_1v8  "IO8_FT_V33 med speed @ 1.8V pullup"
io8_ft_v33_ms_pd_1v8  "IO8_FT_V33 med speed @ 1.8V pulldown"
io8_ft_v33_ls_1v8  "IO8_FT_V33 low speed @ 1.8V"
io8_ft_v33_ls_pu_1v8  "IO8_FT_V33 low speed @ 1.8V pullup"
io8_ft_v33_ls_pd_1v8  "IO8_FT_V33 low speed @ 1.8V pulldown"
io8_ft_v33_hs_3v3  "IO8_FT_V33 high speed @ 3.3V"
io8_ft_v33_hs_pu_3v3  "IO8_FT_V33 high speed @ 3.3V pullup"
io8_ft_v33_hs_pd_3v3  "IO8_FT_V33 high speed @ 3.3V pulldown"
io8_ft_v33_fs_3v3  "IO8_FT_V33 fast speed @ 3.3V"
io8_ft_v33_fs_pu_3v3  "IO8_FT_V33 fast speed @ 3.3V pullup"
io8_ft_v33_fs_pd_3v3  "IO8_FT_V33 fast speed @ 3.3V pulldown"
io8_ft_v33_ms_3v3  "IO8_FT_V33 med speed @ 3.3V"
io8_ft_v33_ms_pu_3v3  "IO8_FT_V33 med speed @ 3.3V pullup"
io8_ft_v33_ms_pd_3v3  "IO8_FT_V33 med speed @ 3.3V pulldown"
io8_ft_v33_ls_3v3  "IO8_FT_V33 low speed @ 3.3V"
io8_ft_v33_ls_pu_3v3  "IO8_FT_V33 low speed @ 3.3V pullup"
io8_ft_v33_ls_pd_3v3  "IO8_FT_V33 low speed @ 3.3V pulldown"
[Model Selector] io8_100m_usb_id
io8_100m_ft_hs_1v2  "IO8_FT 100MHz high speed @ 1.2V"
io8_100m_ft_hs_pu_1v2  "IO8_FT 100MHz high speed @ 1.2V pullup"
io8_100m_ft_hs_pd_1v2  "IO8_FT 100MHz high speed @ 1.2V pulldown"
io8_100m_ft_fs_1v2  "IO8_FT 100MHz fast speed @ 1.2V"
io8_100m_ft_fs_pu_1v2  "IO8_FT 100MHz fast speed @ 1.2V pullup"
io8_100m_ft_fs_pd_1v2  "IO8_FT 100MHz fast speed @ 1.2V pulldown"
io8_100m_ft_ms_1v2  "IO8_FT 100MHz med speed @ 1.2V"
io8_100m_ft_ms_pu_1v2  "IO8_FT 100MHz med speed @ 1.2V pullup"
io8_100m_ft_ms_pd_1v2  "IO8_FT 100MHz med speed @ 1.2V pulldown"
io8_100m_ft_ls_1v2  "IO8_FT 100MHz low speed @ 1.2V"
io8_100m_ft_ls_pu_1v2  "IO8_FT 100MHz low speed @ 1.2V pullup"
io8_100m_ft_ls_pd_1v2  "IO8_FT 100MHz low speed @ 1.2V pulldown"
io8_100m_ft_hs_1v8  "IO8_FT 100MHz high speed @ 1.8V"
io8_100m_ft_hs_pu_1v8  "IO8_FT 100MHz high speed @ 1.8V pullup"
io8_100m_ft_hs_pd_1v8  "IO8_FT 100MHz high speed @ 1.8V pulldown"
io8_100m_ft_fs_1v8  "IO8_FT 100MHz fast speed @ 1.8V"
io8_100m_ft_fs_pu_1v8  "IO8_FT 100MHz fast speed @ 1.8V pullup"
io8_100m_ft_fs_pd_1v8  "IO8_FT 100MHz fast speed @ 1.8V pulldown"
io8_100m_ft_ms_1v8  "IO8_FT 100MHz med speed @ 1.8V"
io8_100m_ft_ms_pu_1v8  "IO8_FT 100MHz med speed @ 1.8V pullup"
io8_100m_ft_ms_pd_1v8  "IO8_FT 100MHz med speed @ 1.8V pulldown"
io8_100m_ft_ls_1v8  "IO8_FT 100MHz low speed @ 1.8V"
io8_100m_ft_ls_pu_1v8  "IO8_FT 100MHz low speed @ 1.8V pullup"
io8_100m_ft_ls_pd_1v8  "IO8_FT 100MHz low speed @ 1.8V pulldown"
io8_100m_ft_hs_3v3  "IO8_FT 100MHz high speed @ 3.3V"
io8_100m_ft_hs_pu_3v3  "IO8_FT 100MHz high speed @ 3.3V pullup"
io8_100m_ft_hs_pd_3v3  "IO8_FT 100MHz high speed @ 3.3V pulldown"
io8_100m_ft_fs_3v3  "IO8_FT 100MHz fast speed @ 3.3V"
io8_100m_ft_fs_pu_3v3  "IO8_FT 100MHz fast speed @ 3.3V pullup"
io8_100m_ft_fs_pd_3v3  "IO8_FT 100MHz fast speed @ 3.3V pulldown"
io8_100m_ft_ms_3v3  "IO8_FT 100MHz med speed @ 3.3V"
io8_100m_ft_ms_pu_3v3  "IO8_FT 100MHz med speed @ 3.3V pullup"
io8_100m_ft_ms_pd_3v3  "IO8_FT 100MHz med speed @ 3.3V pulldown"
io8_100m_ft_ls_3v3  "IO8_FT 100MHz low speed @ 3.3V"
io8_100m_ft_ls_pu_3v3  "IO8_FT 100MHz low speed @ 3.3V pullup"
io8_100m_ft_ls_pd_3v3  "IO8_FT 100MHz low speed @ 3.3V pulldown"
io8usb_id_nopu  "IOUSB ID @ 3.3V"
io8usb_id_pu  "IOUSB ID @ 3.3V pullup"
[Model Selector] io8_100m_usb_vbus_ft
io8_100m_ft_hs_1v2  "IO8_FT 100MHz high speed @ 1.2V"
io8_100m_ft_hs_pu_1v2  "IO8_FT 100MHz high speed @ 1.2V pullup"
io8_100m_ft_hs_pd_1v2  "IO8_FT 100MHz high speed @ 1.2V pulldown"
io8_100m_ft_fs_1v2  "IO8_FT 100MHz fast speed @ 1.2V"
io8_100m_ft_fs_pu_1v2  "IO8_FT 100MHz fast speed @ 1.2V pullup"
io8_100m_ft_fs_pd_1v2  "IO8_FT 100MHz fast speed @ 1.2V pulldown"
io8_100m_ft_ms_1v2  "IO8_FT 100MHz med speed @ 1.2V"
io8_100m_ft_ms_pu_1v2  "IO8_FT 100MHz med speed @ 1.2V pullup"
io8_100m_ft_ms_pd_1v2  "IO8_FT 100MHz med speed @ 1.2V pulldown"
io8_100m_ft_ls_1v2  "IO8_FT 100MHz low speed @ 1.2V"
io8_100m_ft_ls_pu_1v2  "IO8_FT 100MHz low speed @ 1.2V pullup"
io8_100m_ft_ls_pd_1v2  "IO8_FT 100MHz low speed @ 1.2V pulldown"
io8_100m_ft_hs_1v8  "IO8_FT 100MHz high speed @ 1.8V"
io8_100m_ft_hs_pu_1v8  "IO8_FT 100MHz high speed @ 1.8V pullup"
io8_100m_ft_hs_pd_1v8  "IO8_FT 100MHz high speed @ 1.8V pulldown"
io8_100m_ft_fs_1v8  "IO8_FT 100MHz fast speed @ 1.8V"
io8_100m_ft_fs_pu_1v8  "IO8_FT 100MHz fast speed @ 1.8V pullup"
io8_100m_ft_fs_pd_1v8  "IO8_FT 100MHz fast speed @ 1.8V pulldown"
io8_100m_ft_ms_1v8  "IO8_FT 100MHz med speed @ 1.8V"
io8_100m_ft_ms_pu_1v8  "IO8_FT 100MHz med speed @ 1.8V pullup"
io8_100m_ft_ms_pd_1v8  "IO8_FT 100MHz med speed @ 1.8V pulldown"
io8_100m_ft_ls_1v8  "IO8_FT 100MHz low speed @ 1.8V"
io8_100m_ft_ls_pu_1v8  "IO8_FT 100MHz low speed @ 1.8V pullup"
io8_100m_ft_ls_pd_1v8  "IO8_FT 100MHz low speed @ 1.8V pulldown"
io8_100m_ft_hs_3v3  "IO8_FT 100MHz high speed @ 3.3V"
io8_100m_ft_hs_pu_3v3  "IO8_FT 100MHz high speed @ 3.3V pullup"
io8_100m_ft_hs_pd_3v3  "IO8_FT 100MHz high speed @ 3.3V pulldown"
io8_100m_ft_fs_3v3  "IO8_FT 100MHz fast speed @ 3.3V"
io8_100m_ft_fs_pu_3v3  "IO8_FT 100MHz fast speed @ 3.3V pullup"
io8_100m_ft_fs_pd_3v3  "IO8_FT 100MHz fast speed @ 3.3V pulldown"
io8_100m_ft_ms_3v3  "IO8_FT 100MHz med speed @ 3.3V"
io8_100m_ft_ms_pu_3v3  "IO8_FT 100MHz med speed @ 3.3V pullup"
io8_100m_ft_ms_pd_3v3  "IO8_FT 100MHz med speed @ 3.3V pulldown"
io8_100m_ft_ls_3v3  "IO8_FT 100MHz low speed @ 3.3V"
io8_100m_ft_ls_pu_3v3  "IO8_FT 100MHz low speed @ 3.3V pullup"
io8_100m_ft_ls_pd_3v3  "IO8_FT 100MHz low speed @ 3.3V pulldown"
io8usb_adp "IOUSB ADP @ 3.3V"
io8usb_vbus "IOUSB VBUS @ 3.3V"
[Model Selector] io8_usb_ft
io8_100m_ft_hs_1v2  "IO8_FT 100MHz high speed @ 1.2V"
io8_100m_ft_hs_pu_1v2  "IO8_FT 100MHz high speed @ 1.2V pullup"
io8_100m_ft_hs_pd_1v2  "IO8_FT 100MHz high speed @ 1.2V pulldown"
io8_100m_ft_fs_1v2  "IO8_FT 100MHz fast speed @ 1.2V"
io8_100m_ft_fs_pu_1v2  "IO8_FT 100MHz fast speed @ 1.2V pullup"
io8_100m_ft_fs_pd_1v2  "IO8_FT 100MHz fast speed @ 1.2V pulldown"
io8_100m_ft_ms_1v2  "IO8_FT 100MHz med speed @ 1.2V"
io8_100m_ft_ms_pu_1v2  "IO8_FT 100MHz med speed @ 1.2V pullup"
io8_100m_ft_ms_pd_1v2  "IO8_FT 100MHz med speed @ 1.2V pulldown"
io8_100m_ft_ls_1v2  "IO8_FT 100MHz low speed @ 1.2V"
io8_100m_ft_ls_pu_1v2  "IO8_FT 100MHz low speed @ 1.2V pullup"
io8_100m_ft_ls_pd_1v2  "IO8_FT 100MHz low speed @ 1.2V pulldown"
io8_100m_ft_hs_1v8  "IO8_FT 100MHz high speed @ 1.8V"
io8_100m_ft_hs_pu_1v8  "IO8_FT 100MHz high speed @ 1.8V pullup"
io8_100m_ft_hs_pd_1v8  "IO8_FT 100MHz high speed @ 1.8V pulldown"
io8_100m_ft_fs_1v8  "IO8_FT 100MHz fast speed @ 1.8V"
io8_100m_ft_fs_pu_1v8  "IO8_FT 100MHz fast speed @ 1.8V pullup"
io8_100m_ft_fs_pd_1v8  "IO8_FT 100MHz fast speed @ 1.8V pulldown"
io8_100m_ft_ms_1v8  "IO8_FT 100MHz med speed @ 1.8V"
io8_100m_ft_ms_pu_1v8  "IO8_FT 100MHz med speed @ 1.8V pullup"
io8_100m_ft_ms_pd_1v8  "IO8_FT 100MHz med speed @ 1.8V pulldown"
io8_100m_ft_ls_1v8  "IO8_FT 100MHz low speed @ 1.8V"
io8_100m_ft_ls_pu_1v8  "IO8_FT 100MHz low speed @ 1.8V pullup"
io8_100m_ft_ls_pd_1v8  "IO8_FT 100MHz low speed @ 1.8V pulldown"
io8_100m_ft_hs_3v3  "IO8_FT 100MHz high speed @ 3.3V"
io8_100m_ft_hs_pu_3v3  "IO8_FT 100MHz high speed @ 3.3V pullup"
io8_100m_ft_hs_pd_3v3  "IO8_FT 100MHz high speed @ 3.3V pulldown"
io8_100m_ft_fs_3v3  "IO8_FT 100MHz fast speed @ 3.3V"
io8_100m_ft_fs_pu_3v3  "IO8_FT 100MHz fast speed @ 3.3V pullup"
io8_100m_ft_fs_pd_3v3  "IO8_FT 100MHz fast speed @ 3.3V pulldown"
io8_100m_ft_ms_3v3  "IO8_FT 100MHz med speed @ 3.3V"
io8_100m_ft_ms_pu_3v3  "IO8_FT 100MHz med speed @ 3.3V pullup"
io8_100m_ft_ms_pd_3v3  "IO8_FT 100MHz med speed @ 3.3V pulldown"
io8_100m_ft_ls_3v3  "IO8_FT 100MHz low speed @ 3.3V"
io8_100m_ft_ls_pu_3v3  "IO8_FT 100MHz low speed @ 3.3V pullup"
io8_100m_ft_ls_pd_3v3  "IO8_FT 100MHz low speed @ 3.3V pulldown"
io8_usb_fs_3v3  "IOUSB fast speed @ 3.3V"
io8_usb_fs_pu1_3v3  "IO8USB fast speed @ 3.3V pullup1"
io8_usb_fs_pd1_3v3  "IOUSB fast speed @ 3.3V pulldown1"
io8_usb_ls_3v3  "IOUSB low speed @ 3.3V"
io8_usb_ls_pu1_3v3  "IOUSB low speed @ 3.3V pullup1"
io8_usb_ls_pd1_3v3  "IOUSB low speed @ 3.3V pulldown1"
io8_usb_fs_pu2_3v3  "IOUSB fast speed @ 3.3V pullup2"
io8_usb_fs_pd2_3v3  "IOUSB fast speed @ 3.3V pulldown2"
io8_usb_ls_pu2_3v3  "IOUSB low speed @ 3.3V pullup2"
io8_usb_ls_pd2_3v3  "IOUSB low speed @ 3.3V pulldown2"
[Model Selector] io8_100m_i2c_ft
io8_100m_ft_hs_1v2  "IO8_FT 100MHz high speed @ 1.2V"
io8_100m_ft_hs_pu_1v2  "IO8_FT 100MHz high speed @ 1.2V pullup"
io8_100m_ft_hs_pd_1v2  "IO8_FT 100MHz high speed @ 1.2V pulldown"
io8_100m_ft_fs_1v2  "IO8_FT 100MHz fast speed @ 1.2V"
io8_100m_ft_fs_pu_1v2  "IO8_FT 100MHz fast speed @ 1.2V pullup"
io8_100m_ft_fs_pd_1v2  "IO8_FT 100MHz fast speed @ 1.2V pulldown"
io8_100m_ft_ms_1v2  "IO8_FT 100MHz med speed @ 1.2V"
io8_100m_ft_ms_pu_1v2  "IO8_FT 100MHz med speed @ 1.2V pullup"
io8_100m_ft_ms_pd_1v2  "IO8_FT 100MHz med speed @ 1.2V pulldown"
io8_100m_ft_ls_1v2  "IO8_FT 100MHz low speed @ 1.2V"
io8_100m_ft_ls_pu_1v2  "IO8_FT 100MHz low speed @ 1.2V pullup"
io8_100m_ft_ls_pd_1v2  "IO8_FT 100MHz low speed @ 1.2V pulldown"
io8_100m_ft_hs_1v8  "IO8_FT 100MHz high speed @ 1.8V"
io8_100m_ft_hs_pu_1v8  "IO8_FT 100MHz high speed @ 1.8V pullup"
io8_100m_ft_hs_pd_1v8  "IO8_FT 100MHz high speed @ 1.8V pulldown"
io8_100m_ft_fs_1v8  "IO8_FT 100MHz fast speed @ 1.8V"
io8_100m_ft_fs_pu_1v8  "IO8_FT 100MHz fast speed @ 1.8V pullup"
io8_100m_ft_fs_pd_1v8  "IO8_FT 100MHz fast speed @ 1.8V pulldown"
io8_100m_ft_ms_1v8  "IO8_FT 100MHz med speed @ 1.8V"
io8_100m_ft_ms_pu_1v8  "IO8_FT 100MHz med speed @ 1.8V pullup"
io8_100m_ft_ms_pd_1v8  "IO8_FT 100MHz med speed @ 1.8V pulldown"
io8_100m_ft_ls_1v8  "IO8_FT 100MHz low speed @ 1.8V"
io8_100m_ft_ls_pu_1v8  "IO8_FT 100MHz low speed @ 1.8V pullup"
io8_100m_ft_ls_pd_1v8  "IO8_FT 100MHz low speed @ 1.8V pulldown"
io8_100m_ft_hs_3v3  "IO8_FT 100MHz high speed @ 3.3V"
io8_100m_ft_hs_pu_3v3  "IO8_FT 100MHz high speed @ 3.3V pullup"
io8_100m_ft_hs_pd_3v3  "IO8_FT 100MHz high speed @ 3.3V pulldown"
io8_100m_ft_fs_3v3  "IO8_FT 100MHz fast speed @ 3.3V"
io8_100m_ft_fs_pu_3v3  "IO8_FT 100MHz fast speed @ 3.3V pullup"
io8_100m_ft_fs_pd_3v3  "IO8_FT 100MHz fast speed @ 3.3V pulldown"
io8_100m_ft_ms_3v3  "IO8_FT 100MHz med speed @ 3.3V"
io8_100m_ft_ms_pu_3v3  "IO8_FT 100MHz med speed @ 3.3V pullup"
io8_100m_ft_ms_pd_3v3  "IO8_FT 100MHz med speed @ 3.3V pulldown"
io8_100m_ft_ls_3v3  "IO8_FT 100MHz low speed @ 3.3V"
io8_100m_ft_ls_pu_3v3  "IO8_FT 100MHz low speed @ 3.3V pullup"
io8_100m_ft_ls_pd_3v3  "IO8_FT 100MHz low speed @ 3.3V pulldown"
io8_100m_i2c_ft_1v2  "IO8_FT 100MHz I2C @ 1.2V"
io8_100m_i2c_ft_pu_1v2  "IO8_FT 100MHz I2C @ 1.2V pullup"
io8_100m_i2c_ft_pd_1v2  "IO8_FT 100MHz I2C @ 1.2V pulldown"
io8_100m_i2c_ft_1v8  "IO8_FT 100MHz I2C @ 1.8V"
io8_100m_i2c_ft_pu_1v8  "IO8_FT 100MHz I2C @ 1.8V pullup"
io8_100m_i2c_ft_pd_1v8  "IO8_FT 100MHz I2C @ 1,8V pulldown"
io8_100m_i2c_ft_3v3  "IO8_FT 100MHz I2C @ 3.3V"
io8_100m_i2c_ft_pu_3v3  "IO8_FT 100MHz I2C HSLV @ 3.3V pullup"
io8_100m_i2c_ft_pd_3v3  "IO8_FT 100MHz I2C @ 3.3V pulldown"
[Model Selector] io8_166m_hslv_i2c_ft
io8_166m_ft_hs_1v2  "IO8_FT 166MHz high speed @ 1.2V"
io8_166m_ft_hs_pu_1v2  "IO8_FT 166MHz high speed @ 1.2V pullup"
io8_166m_ft_hs_pd_1v2  "IO8_FT 166MHz high speed @ 1.2V pulldown"
io8_166m_ft_fs_1v2  "IO8_FT 166MHz fast speed @ 1.2V"
io8_166m_ft_fs_pu_1v2  "IO8_FT 166MHz fast speed @ 1.2V pullup"
io8_166m_ft_fs_pd_1v2  "IO8_FT 166MHz fast speed @ 1.2V pulldown"
io8_166m_ft_ms_1v2  "IO8_FT 166MHz med speed @ 1.2V"
io8_166m_ft_ms_pu_1v2  "IO8_FT 166MHz med speed @ 1.2V pullup"
io8_166m_ft_ms_pd_1v2  "IO8_FT 166MHz med speed @ 1.2V pulldown"
io8_166m_ft_ls_1v2  "IO8_FT 166MHz low speed @ 1.2V"
io8_166m_ft_ls_pu_1v2  "IO8_FT 166MHz low speed @ 1.2V pullup"
io8_166m_ft_ls_pd_1v2  "IO8_FT 166MHz low speed @ 1.2V pulldown"
io8_166m_ft_hs_1v8  "IO8_FT 166MHz high speed @ 1.8V"
io8_166m_ft_hs_pu_1v8  "IO8_FT 166MHz high speed @ 1.8V pullup"
io8_166m_ft_hs_pd_1v8  "IO8_FT 166MHz high speed @ 1.8V pulldown"
io8_166m_ft_fs_1v8  "IO8_FT 166MHz fast speed @ 1.8V"
io8_166m_ft_fs_pu_1v8  "IO8_FT 166MHz fast speed @ 1.8V pullup"
io8_166m_ft_fs_pd_1v8  "IO8_FT 166MHz fast speed @ 1.8V pulldown"
io8_166m_ft_ms_1v8  "IO8_FT 166MHz med speed @ 1.8V"
io8_166m_ft_ms_pu_1v8  "IO8_FT 166MHz med speed @ 1.8V pullup"
io8_166m_ft_ms_pd_1v8  "IO8_FT 166MHz med speed @ 1.8V pulldown"
io8_166m_ft_ls_1v8  "IO8_FT 166MHz low speed @ 1.8V"
io8_166m_ft_ls_pu_1v8  "IO8_FT 166MHz low speed @ 1.8V pullup"
io8_166m_ft_ls_pd_1v8  "IO8_FT 166MHz low speed @ 1.8V pulldown"
io8_166m_ft_hs_3v3  "IO8_FT 166MHz high speed @ 3.3V"
io8_166m_ft_hs_pu_3v3  "IO8_FT 166MHz high speed @ 3.3V pullup"
io8_166m_ft_hs_pd_3v3  "IO8_FT 166MHz high speed @ 3.3V pulldown"
io8_166m_ft_fs_3v3  "IO8_FT 166MHz fast speed @ 3.3V"
io8_166m_ft_fs_pu_3v3  "IO8_FT 166MHz fast speed @ 3.3V pullup"
io8_166m_ft_fs_pd_3v3  "IO8_FT 166MHz fast speed @ 3.3V pulldown"
io8_166m_ft_ms_3v3  "IO8_FT 166MHz med speed @ 3.3V"
io8_166m_ft_ms_pu_3v3  "IO8_FT 166MHz med speed @ 3.3V pullup"
io8_166m_ft_ms_pd_3v3  "IO8_FT 166MHz med speed @ 3.3V pulldown"
io8_166m_ft_ls_3v3  "IO8_FT 166MHz low speed @ 3.3V"
io8_166m_ft_ls_pu_3v3  "IO8_FT 166MHz low speed @ 3.3V pullup"
io8_166m_ft_ls_pd_3v3  "IO8_FT 166MHz low speed @ 3.3V pulldown"
io8_166m_hslv_ft_hs_1v2  "IO8_FT 166MHz HSLV high speed @ 1.2V"
io8_166m_hslv_ft_hs_pu_1v2  "IO8_FT 166MHz HSLV high speed @ 1.2V pullup"
io8_166m_hslv_ft_hs_pd_1v2  "IO8_FT 166MHz HSLV high speed @ 1.2V pulldown"
io8_166m_hslv_ft_fs_1v2  "IO8_FT 166MHz HSLV fast speed @ 1.2V"
io8_166m_hslv_ft_fs_pu_1v2  "IO8_FT 166MHz HSLV fast speed @ 1.2V pullup"
io8_166m_hslv_ft_fs_pd_1v2  "IO8_FT 166MHz HSLV fast speed @ 1.2V pulldown"
io8_166m_hslv_ft_ms_1v2  "IO8_FT 166MHz HSLV med speed @ 1.2V"
io8_166m_hslv_ft_ms_pu_1v2  "IO8_FT 166MHz HSLV med speed @ 1.2V pullup"
io8_166m_hslv_ft_ms_pd_1v2  "IO8_FT 166MHz HSLV med speed @ 1.2V pulldown"
io8_166m_hslv_ft_ls_1v2  "IO8_FT 166MHz HSLV low speed @ 1.2V"
io8_166m_hslv_ft_ls_pu_1v2  "IO8_FT 166MHz HSLV low speed @ 1.2V pullup"
io8_166m_hslv_ft_ls_pd_1v2  "IO8_FT 166MHz HSLV low speed @ 1.2V pulldown"
io8_166m_hslv_ft_hs_1v8  "IO8_FT 166MHz HSLV high speed @ 1.8V"
io8_166m_hslv_ft_hs_pu_1v8  "IO8_FT 166MHz HSLV high speed @ 1.8V pullup"
io8_166m_hslv_ft_hs_pd_1v8  "IO8_FT 166MHz HSLV high speed @ 1.8V pulldown"
io8_166m_hslv_ft_fs_1v8  "IO8_FT 166MHz HSLV fast speed @ 1.8V"
io8_166m_hslv_ft_fs_pu_1v8  "IO8_FT 166MHz HSLV fast speed @ 1.8V pullup"
io8_166m_hslv_ft_fs_pd_1v8  "IO8_FT 166MHz HSLV fast speed @ 1.8V pulldown"
io8_166m_hslv_ft_ms_1v8  "IO8_FT 166MHz HSLV med speed @ 1.8V"
io8_166m_hslv_ft_ms_pu_1v8  "IO8_FT 166MHz HSLV med speed @ 1.8V pullup"
io8_166m_hslv_ft_ms_pd_1v8  "IO8_FT 166MHz HSLV med speed @ 1.8V pulldown"
io8_166m_hslv_ft_ls_1v8  "IO8_FT 166MHz HSLV low speed @ 1.8V"
io8_166m_hslv_ft_ls_pu_1v8  "IO8_FT 166MHz HSLV low speed @ 1.8V pullup"
io8_166m_hslv_ft_ls_pd_1v8  "IO8_FT 166MHz HSLV low speed @ 1.8V pulldown"
io8_166m_hslv_ft_hs_2v5  "IO8_FT 166MHz HSLV high speed @ 2.5V"
io8_166m_hslv_ft_hs_pu_2v5  "IO8_FT 166MHz HSLV high speed @ 2.5V pullup"
io8_166m_hslv_ft_hs_pd_2v5  "IO8_FT 166MHz HSLV high speed @ 2.5V pulldown"
io8_166m_hslv_ft_fs_2v5  "IO8_FT 166MHz HSLV fast speed @ 2.5V"
io8_166m_hslv_ft_fs_pu_2v5  "IO8_FT 166MHz HSLV fast speed @ 2.5V pullup"
io8_166m_hslv_ft_fs_pd_2v5  "IO8_FT 166MHz HSLV fast speed @ 2.5V pulldown"
io8_166m_hslv_ft_ms_2v5  "IO8_FT 166MHz HSLV med speed @ 2.5V"
io8_166m_hslv_ft_ms_pu_2v5  "IO8_FT 166MHz HSLV med speed @ 2.5V pullup"
io8_166m_hslv_ft_ms_pd_2v5  "IO8_FT 166MHz HSLV med speed @ 2.5V pulldown"
io8_166m_hslv_ft_ls_2v5  "IO8_FT 166MHz HSLV low speed @ 2.5V"
io8_166m_hslv_ft_ls_pu_2v5  "IO8_FT 166MHz HSLV low speed @ 2.5V pullup"
io8_166m_hslv_ft_ls_pd_2v5  "IO8_FT 166MHz HSLV low speed @ 2.5V pulldown"
io8_166m_i2c_ft_1v2  "IO8_FT 166MHz I2C @ 1.2V"
io8_166m_i2c_ft_pu_1v2  "IO8_FT 166MHz I2C @ 1.2V pullup"
io8_166m_i2c_ft_pd_1v2  "IO8_FT 166MHz I2C @ 1.2V pulldown"
io8_166m_i2c_ft_1v8  "IO8_FT 166MHz I2C @ 1.8V"
io8_166m_i2c_ft_pu_1v8  "IO8_FT 166MHz I2C @ 1.8V pullup"
io8_166m_i2c_ft_pd_1v8  "IO8_FT 166MHz I2C @ 1,8V pulldown"
io8_166m_i2c_ft_3v3  "IO8_FT 166MHz I2C @ 3.3V"
io8_166m_i2c_ft_pu_3v3  "IO8_FT 166MHz I2C HSLV @ 3.3V pullup"
io8_166m_i2c_ft_pd_3v3  "IO8_FT 166MHz I2C @ 3.3V pulldown"
| Models and submodels in the file (212): io8_100m_ft_hs_1v2 (I/O), io8_100m_ft_hs_pu_1v2 (I/O), io8_100m_ft_hs_pd_1v2 (I/O), io8_100m_ft_fs_1v2 (I/O), io8_100m_ft_fs_pu_1v2 (I/O), io8_100m_ft_fs_pd_1v2 (I/O), io8_100m_ft_ms_1v2 (I/O), io8_100m_ft_ms_pu_1v2 (I/O), io8_100m_ft_ms_pd_1v2 (I/O), io8_100m_ft_ls_1v2 (I/O), io8_100m_ft_ls_pu_1v2 (I/O), io8_100m_ft_ls_pd_1v2 (I/O), io8_100m_ft_hs_1v8 (I/O), io8_100m_ft_hs_pu_1v8 (I/O), io8_100m_ft_hs_pd_1v8 (I/O), io8_100m_ft_fs_1v8 (I/O), io8_100m_ft_fs_pu_1v8 (I/O), io8_100m_ft_fs_pd_1v8 (I/O), io8_100m_ft_ms_1v8 (I/O), io8_100m_ft_ms_pu_1v8 (I/O), io8_100m_ft_ms_pd_1v8 (I/O), io8_100m_ft_ls_1v8 (I/O), io8_100m_ft_ls_pu_1v8 (I/O), io8_100m_ft_ls_pd_1v8 (I/O), io8_100m_ft_hs_3v3 (I/O), io8_100m_ft_hs_pu_3v3 (I/O), io8_100m_ft_hs_pd_3v3 (I/O), io8_100m_ft_fs_3v3 (I/O), io8_100m_ft_fs_pu_3v3 (I/O), io8_100m_ft_fs_pd_3v3 (I/O), io8_100m_ft_ms_3v3 (I/O), io8_100m_ft_ms_pu_3v3 (I/O), io8_100m_ft_ms_pd_3v3 (I/O), io8_100m_ft_ls_3v3 (I/O), io8_100m_ft_ls_pu_3v3 (I/O), io8_100m_ft_ls_pd_3v3 (I/O), io8_100m_hslv_ft_hs_1v2 (I/O), io8_100m_hslv_ft_hs_pu_1v2 (I/O), io8_100m_hslv_ft_hs_pd_1v2 (I/O), io8_100m_hslv_ft_fs_1v2 (I/O), io8_100m_hslv_ft_fs_pu_1v2 (I/O), io8_100m_hslv_ft_fs_pd_1v2 (I/O), io8_100m_hslv_ft_ms_1v2 (I/O), io8_100m_hslv_ft_ms_pu_1v2 (I/O), io8_100m_hslv_ft_ms_pd_1v2 (I/O), io8_100m_hslv_ft_ls_1v2 (I/O), io8_100m_hslv_ft_ls_pu_1v2 (I/O), io8_100m_hslv_ft_ls_pd_1v2 (I/O), io8_100m_hslv_ft_hs_1v8 (I/O), io8_100m_hslv_ft_hs_pu_1v8 (I/O), io8_100m_hslv_ft_hs_pd_1v8 (I/O), io8_100m_hslv_ft_fs_1v8 (I/O), io8_100m_hslv_ft_fs_pu_1v8 (I/O), io8_100m_hslv_ft_fs_pd_1v8 (I/O), io8_100m_hslv_ft_ms_1v8 (I/O), io8_100m_hslv_ft_ms_pu_1v8 (I/O), io8_100m_hslv_ft_ms_pd_1v8 (I/O), io8_100m_hslv_ft_ls_1v8 (I/O), io8_100m_hslv_ft_ls_pu_1v8 (I/O), io8_100m_hslv_ft_ls_pd_1v8 (I/O), io8_100m_hslv_ft_hs_2v5 (I/O), io8_100m_hslv_ft_hs_pu_2v5 (I/O), io8_100m_hslv_ft_hs_pd_2v5 (I/O), io8_100m_hslv_ft_fs_2v5 (I/O), io8_100m_hslv_ft_fs_pu_2v5 (I/O), io8_100m_hslv_ft_fs_pd_2v5 (I/O), io8_100m_hslv_ft_ms_2v5 (I/O), io8_100m_hslv_ft_ms_pu_2v5 (I/O), io8_100m_hslv_ft_ms_pd_2v5 (I/O), io8_100m_hslv_ft_ls_2v5 (I/O), io8_100m_hslv_ft_ls_pu_2v5 (I/O), io8_100m_hslv_ft_ls_pd_2v5 (I/O), io8_166m_ft_hs_1v2 (I/O), io8_166m_ft_hs_pu_1v2 (I/O), io8_166m_ft_hs_pd_1v2 (I/O), io8_166m_ft_fs_1v2 (I/O), io8_166m_ft_fs_pu_1v2 (I/O), io8_166m_ft_fs_pd_1v2 (I/O), io8_166m_ft_ms_1v2 (I/O), io8_166m_ft_ms_pu_1v2 (I/O)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
